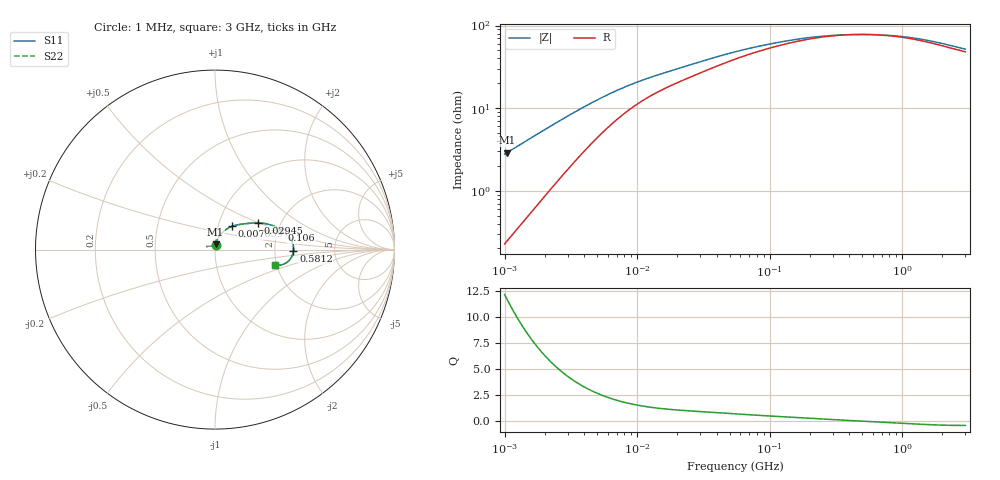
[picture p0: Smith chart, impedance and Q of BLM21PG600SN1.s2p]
! BLM21PG600SN1
# Hz S RI R 50
!Freq.(Hz) S11(Real) S11(Imag) S21(Real) S21(Imag) S12(Real) S12(Imag) S22(Real) S22(Imag)
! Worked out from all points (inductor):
!   401 points, 1 MHz to 3 GHz, reference 50 ohm
!   read as one part in series: L = 438 nH near 1.041 MHz
!   highest Q = 11.7 at 1.041 MHz (marker M1), where L = 440 nH
!   self-resonance near 515.5 MHz
!   S11 on the Smith chart (normalised r, x): 1 MHz: 1.00, +0.06; 7.859 MHz: 1.17, +0.31; 29.45 MHz: 1.53, +0.49; 106 MHz: 2.09, +0.53; 581.2 MHz: 2.55, -0.05; 3 GHz: 1.96, -0.39
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1000000  0.00302 0.0275  0.997 -0.0275  0.997 -0.0275  0.00302 0.0275
1040844  0.00326 0.0286  0.9967 -0.0286  0.9967 -0.0286  0.00326 0.0286
2226959  0.0138 0.0583  0.9862 -0.0583  0.9862 -0.0583  0.0138 0.0583
2947212  0.0229 0.0739  0.9771 -0.0739  0.9771 -0.0739  0.0229 0.0739
3823119  0.0356 0.0901  0.9644 -0.0901  0.9644 -0.0901  0.0356 0.0901
5592179  0.0634 0.1134  0.9366 -0.1134  0.9366 -0.1134  0.0634 0.1134
7858845  0.0963 0.1296  0.9037 -0.1296  0.9037 -0.1296  0.0963 0.1296
1.040059e7  0.1261 0.138  0.8739 -0.138  0.8739 -0.138  0.1261 0.138
1.461624e7  0.1622 0.1437  0.8378 -0.1437  0.8378 -0.1437  0.1622 0.1437
2.944989e7  0.2378 0.1488  0.7622 -0.1488  0.7622 -0.1488  0.2378 0.1488
4.05666e7  0.2749 0.1459  0.7251 -0.1459  0.7251 -0.1459  0.2749 0.1459
5.477226e7  0.3088 0.138  0.6912 -0.138  0.6912 -0.138  0.3088 0.138
7.544761e7  0.3416 0.1252  0.6584 -0.1252  0.6584 -0.1252  0.3416 0.1252
1.060286e8  0.372 0.1083  0.628 -0.1083  0.628 -0.1083  0.372 0.1083
2.094008e8  0.4176 0.0655  0.5824 -0.0655  0.5824 -0.0655  0.4176 0.0655
3.453811e8  0.4346 0.0292  0.5654 -0.0292  0.5654 -0.0292  0.4346 0.0292
5.81181e8  0.4372 -0.0087  0.5628 0.0087  0.5628 0.0087  0.4372 -0.0087
8.005644e8  0.4312 -0.0318  0.5688 0.0318  0.5688 0.0318  0.4312 -0.0318
1.10276e9  0.4183 -0.0541  0.5817 0.0541  0.5817 0.0541  0.4183 -0.0541
1.519029e9  0.3975 -0.0732  0.6025 0.0732  0.6025 0.0732  0.3975 -0.0732
2.134733e9  0.3679 -0.0857  0.6321 0.0857  0.6321 0.0857  0.3679 -0.0857
3e9  0.3357 -0.0867  0.6643 0.0867  0.6643 0.0867  0.3357 -0.0867
